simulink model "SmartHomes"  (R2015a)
settings: Solver=ode45  StartTime=0.0  StopTime=87600  RelTol=1e-3
model workspace (MAT data in the model file):
  batteryCostPerKwh = 500
  batterySize = 7
  oneTimeCost = 1000
  costPerKwhFromUtility = 0.2881
  annualChangeOfCostPerKwhFromUtility = 3.4
  solarPanelEfficiency = 16
  costPerKwhBoughtFromBattery = 0.18
  compensationPerKwhSoldToBattery = 0.18
  numberOfHouses = 1
  MCOS : class17 (value not decoded)
  MCOS : class17 (value not decoded)
undefined symbols (not defined in the file or in its folder): csvread, randi
libraries: simulink x19

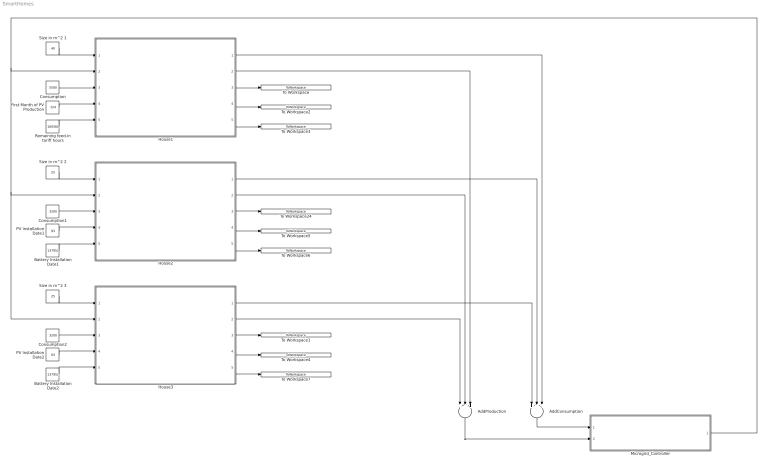
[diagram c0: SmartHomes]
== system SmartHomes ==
  AddConsumption : Sum  Inputs=+++
  AddProduction : Sum  Inputs=+++
  Battery Installation Date1 : Constant  Value=137952
  Battery Installation Date2 : Constant  Value=137952
  Consumption : Constant  Value=5500
  Consumption1 : Constant  Value=3200
  Consumption2 : Constant  Value=3200
  First Month of PV Production : Constant  Value=124
  House1 : Subsystem
  House2 : Subsystem
  House3 : Subsystem
  Microgrid_Controller : Subsystem
  PV Installation Date1 : Constant  Value=93
  PV Installation Date2 : Constant  Value=93
  Remaining feed-in tariff hours : Constant  Value=160560
  Size in m^2 1 : Constant  Value=40
  Size in m^2 2 : Constant  Value=25
  Size in m^2 3 : Constant  Value=25
  To Workspace : ToWorkspace  VariableName=merged_amortisation_house1  SaveFormat=Timeseries  SampleTime=-1
  To Workspace1 : ToWorkspace  VariableName=merged_amortisation_house  SaveFormat=Timeseries  SampleTime=-1
  To Workspace2 : ToWorkspace  VariableName=split_amortisation_house1  SaveFormat=Timeseries  SampleTime=-1
  To Workspace24 : ToWorkspace  VariableName=merged_amortisation_house2  SaveFormat=Timeseries  SampleTime=-1
  To Workspace3 : ToWorkspace  VariableName=net_sale_gradiant_house1  SaveFormat=Timeseries  SampleTime=-1
  To Workspace4 : ToWorkspace  VariableName=split_amortisation_house  SaveFormat=Timeseries  SampleTime=-1
  To Workspace5 : ToWorkspace  VariableName=split_amortisation_house2  SaveFormat=Timeseries  SampleTime=-1
  To Workspace6 : ToWorkspace  VariableName=net_sale_gradiant_house2  SaveFormat=Timeseries  SampleTime=-1
  To Workspace7 : ToWorkspace  VariableName=net_sale_gradiant_house  SaveFormat=Timeseries  SampleTime=-1
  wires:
  Size in m^2 1/1 -> House1/1(Solar Panel Size m²)
  AddConsumption/1 -> Microgrid_Controller/1(Energy Consumption (kWh))
  Consumption/1 -> House1/3(Yearly Consumption (kWh))
  AddProduction/1 -> Microgrid_Controller/2(Energy Production (kWh))
  House1/3(Merged Amortisation) -> To Workspace/1
  House1/4(Split Amortisation) -> To Workspace2/1
  House2/4(Split Amortisation) -> To Workspace5/1
  House2/3(Merged Amortisation) -> To Workspace24/1
  Remaining feed-in tariff hours/1 -> House1/5(Hours of Feed-In Tariff Remaining)
  First Month of PV Production/1 -> House1/4(First Month of PV Production)
  House1/2(Effective Energy Production (kWh)) -> AddProduction/3
  House1/1(Effective Energy Consumption (kWh)) -> AddConsumption/3
  House1/5(Grid Sale Gradient) -> To Workspace3/1
  House2/5(Grid Sale Gradient) -> To Workspace6/1
  Size in m^2 2/1 -> House2/1(Solar Panel Size m²)
  Consumption1/1 -> House2/3(Yearly Consumption (kWh))
  Battery Installation Date1/1 -> House2/5(Hours of Feed-In Tariff Remaining)
  PV Installation Date1/1 -> House2/4(First Month of PV Production)
  House3/4(Split Amortisation) -> To Workspace4/1
  House3/3(Merged Amortisation) -> To Workspace1/1
  House3/5(Grid Sale Gradient) -> To Workspace7/1
  Size in m^2 3/1 -> House3/1(Solar Panel Size m²)
  Consumption2/1 -> House3/3(Yearly Consumption (kWh))
  Battery Installation Date2/1 -> House3/5(Hours of Feed-In Tariff Remaining)
  PV Installation Date2/1 -> House3/4(First Month of PV Production)
  Microgrid_Controller/1(Battery Status) -> House1/2(Battey Status), House3/2(Battey Status), House2/2(Battey Status)
  House2/1(Effective Energy Consumption (kWh)) -> AddConsumption/2
  House2/2(Effective Energy Production (kWh)) -> AddProduction/2
  House3/1(Effective Energy Consumption (kWh)) -> AddConsumption/1
  House3/2(Effective Energy Production (kWh)) -> AddProduction/1

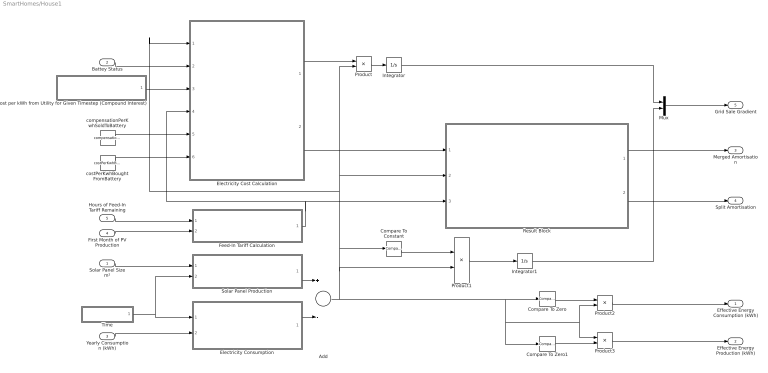
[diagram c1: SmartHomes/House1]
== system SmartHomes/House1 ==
  Solar Panel Size m² : Inport
  Battey Status : Inport  Port=2
  Yearly Consumption (kWh) : Inport  Port=3
  First Month of PV Production : Inport  Port=4
  Hours of Feed-In Tariff Remaining : Inport  Port=5
  Add : Sum  Inputs=+-
  Compare To Constant : simulink/Logic and Bit Operations/Compare To Constant  relop=>=  const=0  OutDataTypeStr=boolean
  Compare To Zero : simulink/Logic and Bit Operations/Compare To Zero  relop=<  OutDataTypeStr=boolean
  Compare To Zero1 : simulink/Logic and Bit Operations/Compare To Zero  relop=>=  OutDataTypeStr=boolean
  Cost per kWh from Utility for Given Timestep (Compound Interest) : Subsystem
  Electricity Consumption : Subsystem
  Electricity Cost Calculation : MATLAB Function  TreatAsAtomicUnit=on
  Feed-In Tariff Calculation : Subsystem
  Integrator : Integrator
  Integrator1 : Integrator
  Mux : Mux  Inputs=2
  Product{,1..3} (4 alike) : Product
  Result Block : Subsystem
  Solar Panel Production : Subsystem
  Time : Subsystem
  compensationPerKwhSoldToBattery : Constant  Value=compensationPerKwhSoldToBattery
  costPerKwhBoughtFromBattery : Constant  Value=costPerKwhBoughtFromBattery
  Effective Energy Consumption (kWh) : Outport
  Effective Energy Production (kWh) : Outport  Port=2
  Merged Amortisation : Outport  Port=3
  Split Amortisation : Outport  Port=4
  Grid Sale Gradient : Outport  Port=5
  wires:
  Time/1(Time in Hours % 8760) -> Solar Panel Production/2(Hour of Year), Electricity Consumption/1(Hour of Year)
  Solar Panel Size m²/1 -> Solar Panel Production/1(Solar Panel Size (m²))
  Yearly Consumption (kWh)/1 -> Electricity Consumption/2(Yearly Consumption (kWh))
  Product/1 -> Integrator/1
  Compare To Constant/1 -> Product1/1
  Product1/1 -> Integrator1/1
  Product2/1 -> Effective Energy Consumption (kWh)/1
  Product3/1 -> Effective Energy Production (kWh)/1
  Compare To Zero1/1 -> Product3/2
  Compare To Zero/1 -> Product2/1
  Battey Status/1 -> Electricity Cost Calculation/2(batteryStatus)
  costPerKwhBoughtFromBattery/1 -> Electricity Cost Calculation/6(internalBuyPrice)
  Cost per kWh from Utility for Given Timestep (Compound Interest)/1(Cost for kWh from Utility at Timestep) -> Electricity Cost Calculation/3(buyPrice)
  Electricity Cost Calculation/1(gridsaleAmount) -> Product/1
  Electricity Consumption/1(Consumtion kWh) -> Add/2
  Solar Panel Production/1(Solar Panel Production (kWh)) -> Add/1
  Add/1 -> Compare To Zero1/1, Product3/1, Product2/2, Compare To Zero/1, Product/2, Result Block/2(Effective Consumption / Production (kWh)), Electricity Cost Calculation/1(kWh), Compare To Constant/1, Product1/2
  Feed-In Tariff Calculation/1(Applcable Feed-In Tariff) -> Electricity Cost Calculation/4(sellPrice), Result Block/3(Applicable Feed-In Tariff (EUR))
  Result Block/1(House Result Merged) -> Merged Amortisation/1
  Result Block/2(House Result Split) -> Split Amortisation/1
  Integrator/1 -> Mux/1
  Integrator1/1 -> Mux/2
  Mux/1 -> Grid Sale Gradient/1
  Electricity Cost Calculation/2(cost) -> Result Block/1(Effective Cost of Electricity for Timestep (EUR))
  Hours of Feed-In Tariff Remaining/1 -> Feed-In Tariff Calculation/1(Hours of Feed-In Tariff Remaining)
  First Month of PV Production/1 -> Feed-In Tariff Calculation/2(First Month of PV Production)
  compensationPerKwhSoldToBattery/1 -> Electricity Cost Calculation/5(internalSellPrice)

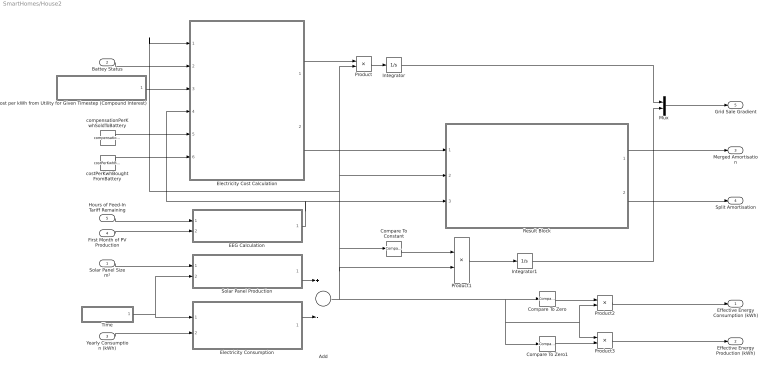
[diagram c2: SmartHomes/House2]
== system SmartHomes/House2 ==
  Solar Panel Size m² : Inport
  Battey Status : Inport  Port=2
  Yearly Consumption (kWh) : Inport  Port=3
  First Month of PV Production : Inport  Port=4
  Hours of Feed-In Tariff Remaining : Inport  Port=5
  Add : Sum  Inputs=+-
  Compare To Constant : simulink/Logic and Bit Operations/Compare To Constant  relop=>=  const=0  OutDataTypeStr=boolean
  Compare To Zero : simulink/Logic and Bit Operations/Compare To Zero  relop=<  OutDataTypeStr=boolean
  Compare To Zero1 : simulink/Logic and Bit Operations/Compare To Zero  relop=>=  OutDataTypeStr=boolean
  Cost per kWh from Utility for Given Timestep (Compound Interest) : Subsystem
  EEG Calculation : Subsystem
  Electricity Consumption : Subsystem
  Electricity Cost Calculation : MATLAB Function  TreatAsAtomicUnit=on
  Integrator : Integrator
  Integrator1 : Integrator
  Mux : Mux  Inputs=2
  Product{,1..3} (4 alike) : Product
  Result Block : Subsystem
  Solar Panel Production : Subsystem
  Time : Subsystem
  compensationPerKwhSoldToBattery : Constant  Value=compensationPerKwhSoldToBattery
  costPerKwhBoughtFromBattery : Constant  Value=costPerKwhBoughtFromBattery
  Effective Energy Consumption (kWh) : Outport
  Effective Energy Production (kWh) : Outport  Port=2
  Merged Amortisation : Outport  Port=3
  Split Amortisation : Outport  Port=4
  Grid Sale Gradient : Outport  Port=5
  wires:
  Time/1(Time in Hours % 8760) -> Solar Panel Production/2(Hour of Year), Electricity Consumption/1(Hour of Year)
  Solar Panel Size m²/1 -> Solar Panel Production/1(Solar Panel Size (m²))
  Yearly Consumption (kWh)/1 -> Electricity Consumption/2(Yearly Consumption (kWh))
  Product/1 -> Integrator/1
  Compare To Constant/1 -> Product1/1
  Product1/1 -> Integrator1/1
  Product2/1 -> Effective Energy Consumption (kWh)/1
  Product3/1 -> Effective Energy Production (kWh)/1
  Compare To Zero1/1 -> Product3/2
  Compare To Zero/1 -> Product2/1
  Battey Status/1 -> Electricity Cost Calculation/2(batteryStatus)
  costPerKwhBoughtFromBattery/1 -> Electricity Cost Calculation/6(internalBuyPrice)
  Cost per kWh from Utility for Given Timestep (Compound Interest)/1(Cost for kWh from Utility at Timestep) -> Electricity Cost Calculation/3(buyPrice)
  Electricity Cost Calculation/1(gridsaleAmount) -> Product/1
  Electricity Consumption/1(Consumtion kWh) -> Add/2
  Solar Panel Production/1(Solar Panel Production (kWh)) -> Add/1
  Add/1 -> Compare To Zero1/1, Product3/1, Product2/2, Compare To Zero/1, Product/2, Result Block/2(Effective Consumption / Production (kWh)), Electricity Cost Calculation/1(kWh), Compare To Constant/1, Product1/2
  EEG Calculation/1(Applcable Feed-In Tariff) -> Electricity Cost Calculation/4(sellPrice), Result Block/3(Applicable Feed-In Tariff (EUR))
  Result Block/1(House Result Merged) -> Merged Amortisation/1
  Result Block/2(House Result Split) -> Split Amortisation/1
  Integrator/1 -> Mux/1
  Integrator1/1 -> Mux/2
  Mux/1 -> Grid Sale Gradient/1
  Electricity Cost Calculation/2(cost) -> Result Block/1(Effective Cost of Electricity for Timestep (EUR))
  Hours of Feed-In Tariff Remaining/1 -> EEG Calculation/1(Hours of Feed-In Tariff Remaining)
  First Month of PV Production/1 -> EEG Calculation/2(First Month of PV Production)
  compensationPerKwhSoldToBattery/1 -> Electricity Cost Calculation/5(internalSellPrice)

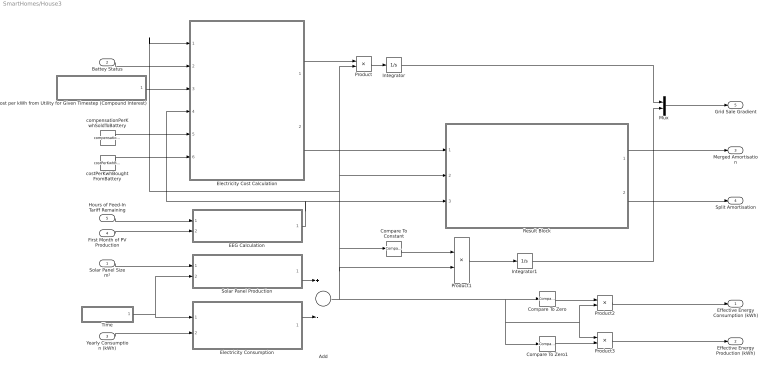
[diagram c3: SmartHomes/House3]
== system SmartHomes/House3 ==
  Solar Panel Size m² : Inport
  Battey Status : Inport  Port=2
  Yearly Consumption (kWh) : Inport  Port=3
  First Month of PV Production : Inport  Port=4
  Hours of Feed-In Tariff Remaining : Inport  Port=5
  Add : Sum  Inputs=+-
  Compare To Constant : simulink/Logic and Bit Operations/Compare To Constant  relop=>=  const=0  OutDataTypeStr=boolean
  Compare To Zero : simulink/Logic and Bit Operations/Compare To Zero  relop=<  OutDataTypeStr=boolean
  Compare To Zero1 : simulink/Logic and Bit Operations/Compare To Zero  relop=>=  OutDataTypeStr=boolean
  Cost per kWh from Utility for Given Timestep (Compound Interest) : Subsystem
  EEG Calculation : Subsystem
  Electricity Consumption : Subsystem
  Electricity Cost Calculation : MATLAB Function  TreatAsAtomicUnit=on
  Integrator : Integrator
  Integrator1 : Integrator
  Mux : Mux  Inputs=2
  Product{,1..3} (4 alike) : Product
  Result Block : Subsystem
  Solar Panel Production : Subsystem
  Time : Subsystem
  compensationPerKwhSoldToBattery : Constant  Value=compensationPerKwhSoldToBattery
  costPerKwhBoughtFromBattery : Constant  Value=costPerKwhBoughtFromBattery
  Effective Energy Consumption (kWh) : Outport
  Effective Energy Production (kWh) : Outport  Port=2
  Merged Amortisation : Outport  Port=3
  Split Amortisation : Outport  Port=4
  Grid Sale Gradient : Outport  Port=5
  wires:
  Time/1(Time in Hours % 8760) -> Solar Panel Production/2(Hour of Year), Electricity Consumption/1(Hour of Year)
  Solar Panel Size m²/1 -> Solar Panel Production/1(Solar Panel Size (m²))
  Yearly Consumption (kWh)/1 -> Electricity Consumption/2(Yearly Consumption (kWh))
  Product/1 -> Integrator/1
  Compare To Constant/1 -> Product1/1
  Product1/1 -> Integrator1/1
  Product2/1 -> Effective Energy Consumption (kWh)/1
  Product3/1 -> Effective Energy Production (kWh)/1
  Compare To Zero1/1 -> Product3/2
  Compare To Zero/1 -> Product2/1
  Battey Status/1 -> Electricity Cost Calculation/2(batteryStatus)
  costPerKwhBoughtFromBattery/1 -> Electricity Cost Calculation/6(internalBuyPrice)
  Cost per kWh from Utility for Given Timestep (Compound Interest)/1(Cost for kWh from Utility at Timestep) -> Electricity Cost Calculation/3(buyPrice)
  Electricity Cost Calculation/1(gridsaleAmount) -> Product/1
  Electricity Consumption/1(Consumtion kWh) -> Add/2
  Solar Panel Production/1(Solar Panel Production (kWh)) -> Add/1
  Add/1 -> Compare To Zero1/1, Product3/1, Product2/2, Compare To Zero/1, Product/2, Result Block/2(Effective Consumption / Production (kWh)), Electricity Cost Calculation/1(kWh), Compare To Constant/1, Product1/2
  EEG Calculation/1(Applcable Feed-In Tariff) -> Electricity Cost Calculation/4(sellPrice), Result Block/3(Applicable Feed-In Tariff (EUR))
  Result Block/1(House Result Merged) -> Merged Amortisation/1
  Result Block/2(House Result Split) -> Split Amortisation/1
  Integrator/1 -> Mux/1
  Integrator1/1 -> Mux/2
  Mux/1 -> Grid Sale Gradient/1
  Electricity Cost Calculation/2(cost) -> Result Block/1(Effective Cost of Electricity for Timestep (EUR))
  Hours of Feed-In Tariff Remaining/1 -> EEG Calculation/1(Hours of Feed-In Tariff Remaining)
  First Month of PV Production/1 -> EEG Calculation/2(First Month of PV Production)
  compensationPerKwhSoldToBattery/1 -> Electricity Cost Calculation/5(internalSellPrice)

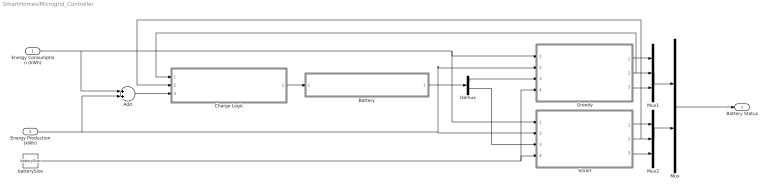
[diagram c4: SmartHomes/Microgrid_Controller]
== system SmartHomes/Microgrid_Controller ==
  Energy Consumption (kWh) : Inport
  Energy Production (kWh) : Inport  Port=2
  Add : Sum
  Battery : Subsystem
  Charge Logic : Subsystem
  Demux : Demux  Outputs=2
  Greedy : MATLAB Function  TreatAsAtomicUnit=on
  Mux : Mux  Inputs=2
  Mux1 : Mux  Inputs=3
  Mux2 : Mux  Inputs=3
  Smart : MATLAB Function  TreatAsAtomicUnit=on
  batterySize : Constant  Value=batterySize
  Battery Status : Outport
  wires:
  Charge Logic/1(Charge (kw/h)) -> Battery/1(Charge Amount (kWh))
  Mux/1 -> Battery Status/1
  batterySize/1 -> Smart/4(batterySize), Greedy/4(batterySize)
  Add/1 -> Charge Logic/3(Net Energy Amount (kWh))
  Demux/2 -> Smart/3(currentBatteryCharge)
  Demux/1 -> Greedy/3(currentBatteryCharge)
  Energy Consumption (kWh)/1 -> Greedy/1(Consumption), Smart/1(Consumption), Add/1
  Energy Production (kWh)/1 -> Smart/2(Production), Greedy/2(Production), Add/2
  Greedy/2(p2) -> Mux1/2, Charge Logic/1(Internal Trade Percentage - Greedy)
  Greedy/3(p3) -> Mux1/3
  Greedy/1(p1) -> Mux1/1
  Mux1/1 -> Mux/1
  Smart/1(p1) -> Mux2/1
  Smart/2(p2) -> Charge Logic/2(Internal Trade Percentage - Smart), Mux2/2
  Smart/3(p3) -> Mux2/3
  Mux2/1 -> Mux/2
  Battery/1(Current Battery Charge (kWh)) -> Demux/1

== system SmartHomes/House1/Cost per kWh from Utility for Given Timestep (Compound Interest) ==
  Calculate Year of Simulation Step : Subsystem
  Compound Interest for Cost per kWh from Utility (EUR) : Fcn  Expr=u(2) * (1 + u(3) / 100) ^ u(1)
  Mux1 : Mux  Inputs=3
  annualChangeOfCostPerKwhFromUtility : Constant  Value=annualChangeOfCostPerKwhFromUtility
  costPerKwhFromUtility : Constant  Value=costPerKwhFromUtility
  Cost for kWh from Utility at Timestep : Outport
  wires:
  Mux1/1 -> Compound Interest for Cost per kWh from Utility (EUR)/1
  annualChangeOfCostPerKwhFromUtility/1 -> Mux1/3
  Calculate Year of Simulation Step/1(Out1) -> Mux1/1
  Compound Interest for Cost per kWh from Utility (EUR)/1 -> Cost for kWh from Utility at Timestep/1
  costPerKwhFromUtility/1 -> Mux1/2

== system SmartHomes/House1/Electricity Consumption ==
  Hour of Year : Inport
  Yearly Consumption (kWh) : Inport  Port=2
  Add : Sum
  Consumption per Hour of Day (kWh) : LookupNDDirect  NumberOfTableDimensions=1  Table=csvread('raw_data/netherlands_consumption_e1a.csv');  DiagnosticForOutOfRangeInput=Error
  Product : Product
  Saturation : Saturate  UpperLimit=5*10e-5  LowerLimit=-5*10e-5
  Variance : RandomNumber  Variance=0.00000000013014  Seed=randi(66666);  SampleTime=1
  Consumtion kWh : Outport
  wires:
  Add/1 -> Product/1
  Consumption per Hour of Day (kWh)/1 -> Add/1
  Hour of Year/1 -> Consumption per Hour of Day (kWh)/1
  Yearly Consumption (kWh)/1 -> Product/2
  Product/1 -> Consumtion kWh/1
  Variance/1 -> Saturation/1
  Saturation/1 -> Add/2

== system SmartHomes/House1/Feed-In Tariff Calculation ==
  Hours of Feed-In Tariff Remaining : Inport
  First Month of PV Production : Inport  Port=2
  Compare To Constant : simulink/Logic and Bit Operations/Compare To Constant  relop=>=  const=0  OutDataTypeStr=boolean
  Constant : Constant  Value=100
  Digtal Clock : DigitalClock
  Divide : Product  Inputs=*/
  EEG-Values : LookupNDDirect  NumberOfTableDimensions=1  Table=csvread('raw_data/feed-in_tariff_data.csv');  DiagnosticForOutOfRangeInput=Error
  Product : Product
  Subtract : Sum  Inputs=+-
  Applcable Feed-In Tariff : Outport
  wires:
  First Month of PV Production/1 -> EEG-Values/1
  Hours of Feed-In Tariff Remaining/1 -> Subtract/1
  Digtal Clock/1 -> Subtract/2
  Subtract/1 -> Compare To Constant/1
  Compare To Constant/1 -> Product/1
  EEG-Values/1 -> Product/2
  Divide/1 -> Applcable Feed-In Tariff/1
  Product/1 -> Divide/1
  Constant/1 -> Divide/2

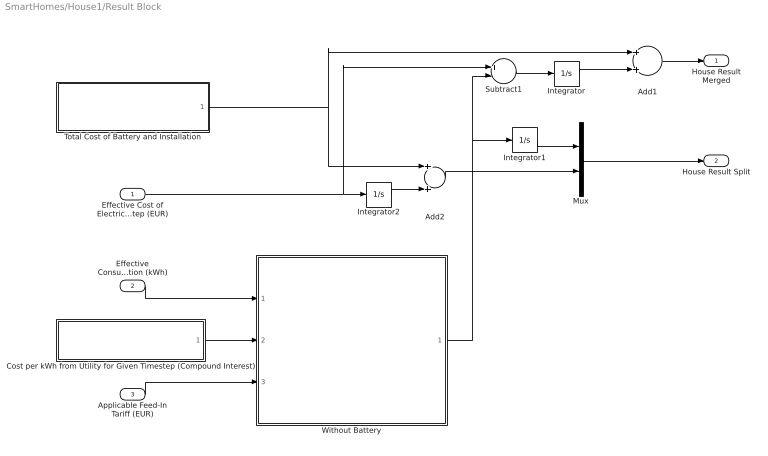
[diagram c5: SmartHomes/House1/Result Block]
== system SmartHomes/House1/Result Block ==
  Effective Cost of Electricity for Timestep (EUR) : Inport
  Effective Consumption / Production (kWh) : Inport  Port=2
  Applicable Feed-In Tariff (EUR) : Inport  Port=3
  Add1 : Sum
  Add2 : Sum
  Cost per kWh from Utility for Given Timestep (Compound Interest) : Subsystem
  Integrator : Integrator
  Integrator1 : Integrator
  Integrator2 : Integrator
  Mux : Mux  Inputs=2
  Subtract1 : Sum  Inputs=+-
  Total Cost of Battery and Installation : Subsystem
  Without Battery : Subsystem
  House Result Merged : Outport
  House Result Split : Outport  Port=2
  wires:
  Applicable Feed-In Tariff (EUR)/1 -> Without Battery/3(Sell Price to Utility (EUR))
  Subtract1/1 -> Integrator/1
  Effective Cost of Electricity for Timestep (EUR)/1 -> Subtract1/1, Integrator2/1
  Add1/1 -> House Result Merged/1
  Effective Consumption / Production (kWh)/1 -> Without Battery/1(Effective Consumption / Production (kWh))
  Integrator/1 -> Add1/2
  Mux/1 -> House Result Split/1
  Integrator1/1 -> Mux/1
  Integrator2/1 -> Add2/2
  Add2/1 -> Mux/2
  Total Cost of Battery and Installation/1(Total Cost of Battery and Installation) -> Add1/1, Add2/1
  Cost per kWh from Utility for Given Timestep (Compound Interest)/1(Cost per kWh from Utility at Timestep) -> Without Battery/2(Cost per kWh from Utility (EUR))
  Without Battery/1(Result EUR) -> Integrator1/1, Subtract1/2

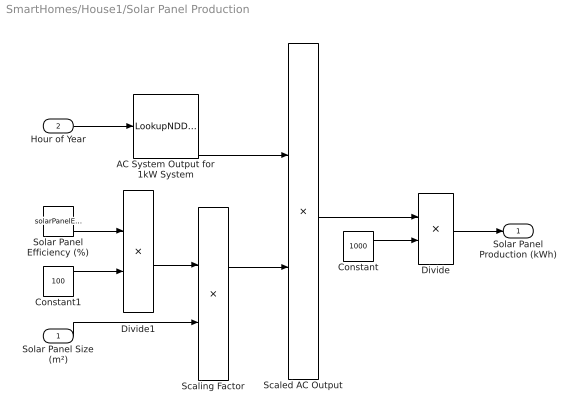
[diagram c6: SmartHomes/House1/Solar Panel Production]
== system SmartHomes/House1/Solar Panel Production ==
  Solar Panel Size (m²) : Inport
  Hour of Year : Inport  Port=2
  AC System Output for 1kW System : LookupNDDirect  NumberOfTableDimensions=1  Table=csvread('raw_data/pvwatts_data_1kwp.csv');  DiagnosticForOutOfRangeInput=Error
  Constant : Constant  Value=1000
  Constant1 : Constant  Value=100
  Divide : Product  Inputs=*/
  Divide1 : Product  Inputs=*/
  Scaled AC Output : Product
  Scaling Factor : Product
  Solar Panel Efficiency (%) : Constant  Value=solarPanelEfficiency
  Solar Panel Production (kWh) : Outport
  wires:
  Solar Panel Efficiency (%)/1 -> Divide1/1
  Scaling Factor/1 -> Scaled AC Output/2
  AC System Output for 1kW System/1 -> Scaled AC Output/1
  Solar Panel Size (m²)/1 -> Scaling Factor/2
  Hour of Year/1 -> AC System Output for 1kW System/1
  Scaled AC Output/1 -> Divide/1
  Constant/1 -> Divide/2
  Divide/1 -> Solar Panel Production (kWh)/1
  Constant1/1 -> Divide1/2
  Divide1/1 -> Scaling Factor/1

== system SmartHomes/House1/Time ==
  Digtal Clock : DigitalClock
  Hours in a Year : Constant  Value=8760
  Modulo : Math  Operator=mod
  Time in Hours % 8760 : Outport
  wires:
  Digtal Clock/1 -> Modulo/1
  Hours in a Year/1 -> Modulo/2
  Modulo/1 -> Time in Hours % 8760/1

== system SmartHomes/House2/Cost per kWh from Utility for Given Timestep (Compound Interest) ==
  Calculate Year of Simulation Step : Subsystem
  Compound Interest for Cost per kWh from Utility (EUR) : Fcn  Expr=u(2) * (1 + u(3) / 100) ^ u(1)
  Mux1 : Mux  Inputs=3
  annualChangeOfCostPerKwhFromUtility : Constant  Value=annualChangeOfCostPerKwhFromUtility
  costPerKwhFromUtility : Constant  Value=costPerKwhFromUtility
  Cost for kWh from Utility at Timestep : Outport
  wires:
  Mux1/1 -> Compound Interest for Cost per kWh from Utility (EUR)/1
  annualChangeOfCostPerKwhFromUtility/1 -> Mux1/3
  Calculate Year of Simulation Step/1(Out1) -> Mux1/1
  Compound Interest for Cost per kWh from Utility (EUR)/1 -> Cost for kWh from Utility at Timestep/1
  costPerKwhFromUtility/1 -> Mux1/2

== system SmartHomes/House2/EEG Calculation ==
  Hours of Feed-In Tariff Remaining : Inport
  First Month of PV Production : Inport  Port=2
  Compare To Constant : simulink/Logic and Bit Operations/Compare To Constant  relop=>=  const=0  OutDataTypeStr=boolean
  Constant : Constant  Value=100
  Digtal Clock : DigitalClock
  Divide : Product  Inputs=*/
  EEG-Values : LookupNDDirect  NumberOfTableDimensions=1  Table=csvread('raw_data/feed-in_tariff_data.csv');  DiagnosticForOutOfRangeInput=Error
  Product : Product
  Subtract : Sum  Inputs=+-
  Applcable Feed-In Tariff : Outport
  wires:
  First Month of PV Production/1 -> EEG-Values/1
  Hours of Feed-In Tariff Remaining/1 -> Subtract/1
  Digtal Clock/1 -> Subtract/2
  Subtract/1 -> Compare To Constant/1
  Compare To Constant/1 -> Product/1
  EEG-Values/1 -> Product/2
  Divide/1 -> Applcable Feed-In Tariff/1
  Product/1 -> Divide/1
  Constant/1 -> Divide/2

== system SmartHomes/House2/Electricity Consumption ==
  Hour of Year : Inport
  Yearly Consumption (kWh) : Inport  Port=2
  Add : Sum
  Consumption per Hour of Day (kWh) : LookupNDDirect  NumberOfTableDimensions=1  Table=csvread('raw_data/netherlands_consumption_e1a.csv');  DiagnosticForOutOfRangeInput=Error
  Product : Product
  Saturation : Saturate  UpperLimit=5*10e-5  LowerLimit=-5*10e-5
  Variance : RandomNumber  Variance=0.00000000013014  Seed=randi(66666);  SampleTime=1
  Consumtion kWh : Outport
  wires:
  Add/1 -> Product/1
  Consumption per Hour of Day (kWh)/1 -> Add/1
  Hour of Year/1 -> Consumption per Hour of Day (kWh)/1
  Yearly Consumption (kWh)/1 -> Product/2
  Product/1 -> Consumtion kWh/1
  Variance/1 -> Saturation/1
  Saturation/1 -> Add/2

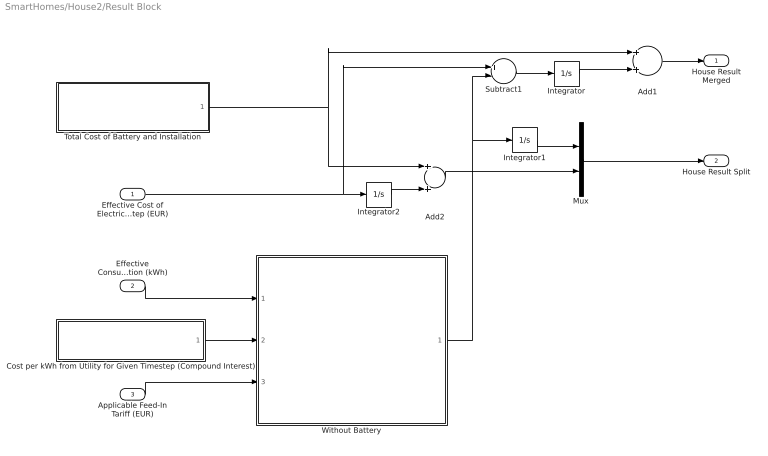
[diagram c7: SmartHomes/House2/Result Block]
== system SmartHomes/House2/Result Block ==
  Effective Cost of Electricity for Timestep (EUR) : Inport
  Effective Consumption / Production (kWh) : Inport  Port=2
  Applicable Feed-In Tariff (EUR) : Inport  Port=3
  Add1 : Sum
  Add2 : Sum
  Cost per kWh from Utility for Given Timestep (Compound Interest) : Subsystem
  Integrator : Integrator
  Integrator1 : Integrator
  Integrator2 : Integrator
  Mux : Mux  Inputs=2
  Subtract1 : Sum  Inputs=+-
  Total Cost of Battery and Installation : Subsystem
  Without Battery : Subsystem
  House Result Merged : Outport
  House Result Split : Outport  Port=2
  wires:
  Applicable Feed-In Tariff (EUR)/1 -> Without Battery/3(Sell Price to Utility (EUR))
  Subtract1/1 -> Integrator/1
  Effective Cost of Electricity for Timestep (EUR)/1 -> Subtract1/1, Integrator2/1
  Add1/1 -> House Result Merged/1
  Effective Consumption / Production (kWh)/1 -> Without Battery/1(Effective Consumption / Production (kWh))
  Integrator/1 -> Add1/2
  Mux/1 -> House Result Split/1
  Integrator1/1 -> Mux/1
  Integrator2/1 -> Add2/2
  Add2/1 -> Mux/2
  Total Cost of Battery and Installation/1(Total Cost of Battery and Installation) -> Add1/1, Add2/1
  Cost per kWh from Utility for Given Timestep (Compound Interest)/1(Cost per kWh from Utility at Timestep) -> Without Battery/2(Cost per kWh from Utility (EUR))
  Without Battery/1(Result EUR) -> Integrator1/1, Subtract1/2

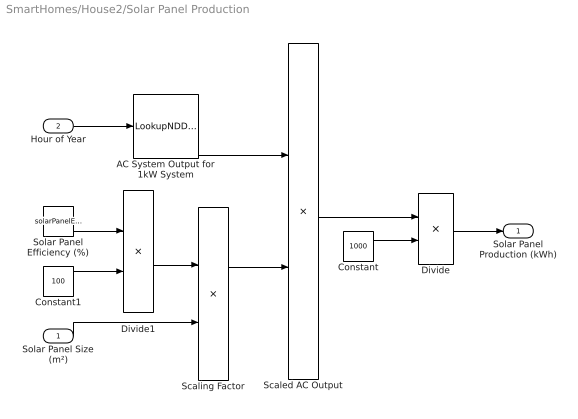
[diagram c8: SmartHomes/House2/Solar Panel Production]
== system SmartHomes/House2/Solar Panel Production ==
  Solar Panel Size (m²) : Inport
  Hour of Year : Inport  Port=2
  AC System Output for 1kW System : LookupNDDirect  NumberOfTableDimensions=1  Table=csvread('raw_data/pvwatts_data_1kwp.csv');  DiagnosticForOutOfRangeInput=Error
  Constant : Constant  Value=1000
  Constant1 : Constant  Value=100
  Divide : Product  Inputs=*/
  Divide1 : Product  Inputs=*/
  Scaled AC Output : Product
  Scaling Factor : Product
  Solar Panel Efficiency (%) : Constant  Value=solarPanelEfficiency
  Solar Panel Production (kWh) : Outport
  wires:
  Solar Panel Efficiency (%)/1 -> Divide1/1
  Scaling Factor/1 -> Scaled AC Output/2
  AC System Output for 1kW System/1 -> Scaled AC Output/1
  Solar Panel Size (m²)/1 -> Scaling Factor/2
  Hour of Year/1 -> AC System Output for 1kW System/1
  Scaled AC Output/1 -> Divide/1
  Constant/1 -> Divide/2
  Divide/1 -> Solar Panel Production (kWh)/1
  Constant1/1 -> Divide1/2
  Divide1/1 -> Scaling Factor/1

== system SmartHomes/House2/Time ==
  Digtal Clock : DigitalClock
  Hours in a Year : Constant  Value=8760
  Modulo : Math  Operator=mod
  Time in Hours % 8760 : Outport
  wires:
  Digtal Clock/1 -> Modulo/1
  Hours in a Year/1 -> Modulo/2
  Modulo/1 -> Time in Hours % 8760/1

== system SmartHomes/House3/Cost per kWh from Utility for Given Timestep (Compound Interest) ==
  Calculate Year of Simulation Step : Subsystem
  Compound Interest for Cost per kWh from Utility (EUR) : Fcn  Expr=u(2) * (1 + u(3) / 100) ^ u(1)
  Mux1 : Mux  Inputs=3
  annualChangeOfCostPerKwhFromUtility : Constant  Value=annualChangeOfCostPerKwhFromUtility
  costPerKwhFromUtility : Constant  Value=costPerKwhFromUtility
  Cost for kWh from Utility at Timestep : Outport
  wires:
  Mux1/1 -> Compound Interest for Cost per kWh from Utility (EUR)/1
  annualChangeOfCostPerKwhFromUtility/1 -> Mux1/3
  Calculate Year of Simulation Step/1(Out1) -> Mux1/1
  Compound Interest for Cost per kWh from Utility (EUR)/1 -> Cost for kWh from Utility at Timestep/1
  costPerKwhFromUtility/1 -> Mux1/2

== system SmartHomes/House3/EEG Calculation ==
  Hours of Feed-In Tariff Remaining : Inport
  First Month of PV Production : Inport  Port=2
  Compare To Constant : simulink/Logic and Bit Operations/Compare To Constant  relop=>=  const=0  OutDataTypeStr=boolean
  Constant : Constant  Value=100
  Digtal Clock : DigitalClock
  Divide : Product  Inputs=*/
  EEG-Values : LookupNDDirect  NumberOfTableDimensions=1  Table=csvread('raw_data/feed-in_tariff_data.csv');  DiagnosticForOutOfRangeInput=Error
  Product : Product
  Subtract : Sum  Inputs=+-
  Applcable Feed-In Tariff : Outport
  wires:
  First Month of PV Production/1 -> EEG-Values/1
  Hours of Feed-In Tariff Remaining/1 -> Subtract/1
  Digtal Clock/1 -> Subtract/2
  Subtract/1 -> Compare To Constant/1
  Compare To Constant/1 -> Product/1
  EEG-Values/1 -> Product/2
  Divide/1 -> Applcable Feed-In Tariff/1
  Product/1 -> Divide/1
  Constant/1 -> Divide/2

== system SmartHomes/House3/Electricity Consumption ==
  Hour of Year : Inport
  Yearly Consumption (kWh) : Inport  Port=2
  Add : Sum
  Consumption per Hour of Day (kWh) : LookupNDDirect  NumberOfTableDimensions=1  Table=csvread('raw_data/netherlands_consumption_e1a.csv');  DiagnosticForOutOfRangeInput=Error
  Product : Product
  Saturation : Saturate  UpperLimit=5*10e-5  LowerLimit=-5*10e-5
  Variance : RandomNumber  Variance=0.00000000013014  Seed=randi(66666);  SampleTime=1
  Consumtion kWh : Outport
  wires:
  Add/1 -> Product/1
  Consumption per Hour of Day (kWh)/1 -> Add/1
  Hour of Year/1 -> Consumption per Hour of Day (kWh)/1
  Yearly Consumption (kWh)/1 -> Product/2
  Product/1 -> Consumtion kWh/1
  Variance/1 -> Saturation/1
  Saturation/1 -> Add/2

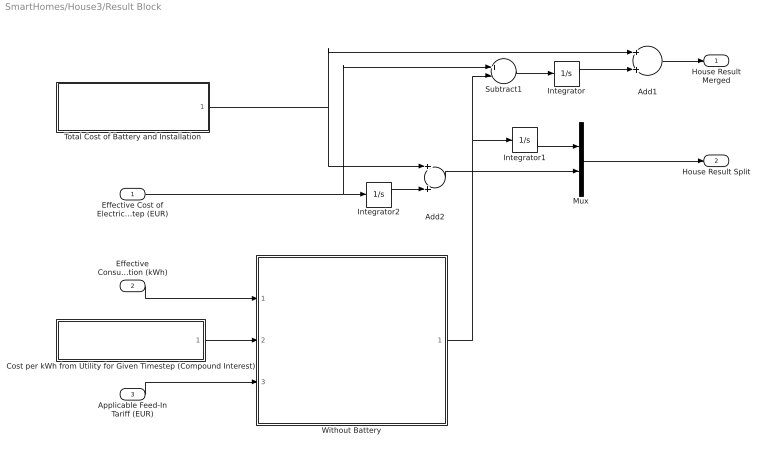
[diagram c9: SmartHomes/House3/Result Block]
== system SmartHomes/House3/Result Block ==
  Effective Cost of Electricity for Timestep (EUR) : Inport
  Effective Consumption / Production (kWh) : Inport  Port=2
  Applicable Feed-In Tariff (EUR) : Inport  Port=3
  Add1 : Sum
  Add2 : Sum
  Cost per kWh from Utility for Given Timestep (Compound Interest) : Subsystem
  Integrator : Integrator
  Integrator1 : Integrator
  Integrator2 : Integrator
  Mux : Mux  Inputs=2
  Subtract1 : Sum  Inputs=+-
  Total Cost of Battery and Installation : Subsystem
  Without Battery : Subsystem
  House Result Merged : Outport
  House Result Split : Outport  Port=2
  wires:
  Applicable Feed-In Tariff (EUR)/1 -> Without Battery/3(Sell Price to Utility (EUR))
  Subtract1/1 -> Integrator/1
  Effective Cost of Electricity for Timestep (EUR)/1 -> Subtract1/1, Integrator2/1
  Add1/1 -> House Result Merged/1
  Effective Consumption / Production (kWh)/1 -> Without Battery/1(Effective Consumption / Production (kWh))
  Integrator/1 -> Add1/2
  Mux/1 -> House Result Split/1
  Integrator1/1 -> Mux/1
  Integrator2/1 -> Add2/2
  Add2/1 -> Mux/2
  Total Cost of Battery and Installation/1(Total Cost of Battery and Installation) -> Add1/1, Add2/1
  Cost per kWh from Utility for Given Timestep (Compound Interest)/1(Cost per kWh from Utility at Timestep) -> Without Battery/2(Cost per kWh from Utility (EUR))
  Without Battery/1(Result EUR) -> Integrator1/1, Subtract1/2

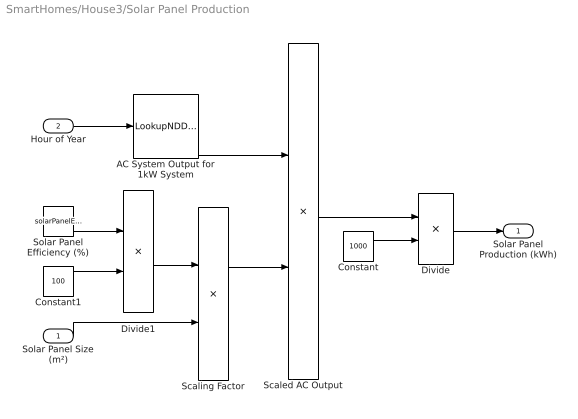
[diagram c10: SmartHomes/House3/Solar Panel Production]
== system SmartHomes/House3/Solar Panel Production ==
  Solar Panel Size (m²) : Inport
  Hour of Year : Inport  Port=2
  AC System Output for 1kW System : LookupNDDirect  NumberOfTableDimensions=1  Table=csvread('raw_data/pvwatts_data_1kwp.csv');  DiagnosticForOutOfRangeInput=Error
  Constant : Constant  Value=1000
  Constant1 : Constant  Value=100
  Divide : Product  Inputs=*/
  Divide1 : Product  Inputs=*/
  Scaled AC Output : Product
  Scaling Factor : Product
  Solar Panel Efficiency (%) : Constant  Value=solarPanelEfficiency
  Solar Panel Production (kWh) : Outport
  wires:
  Solar Panel Efficiency (%)/1 -> Divide1/1
  Scaling Factor/1 -> Scaled AC Output/2
  AC System Output for 1kW System/1 -> Scaled AC Output/1
  Solar Panel Size (m²)/1 -> Scaling Factor/2
  Hour of Year/1 -> AC System Output for 1kW System/1
  Scaled AC Output/1 -> Divide/1
  Constant/1 -> Divide/2
  Divide/1 -> Solar Panel Production (kWh)/1
  Constant1/1 -> Divide1/2
  Divide1/1 -> Scaling Factor/1

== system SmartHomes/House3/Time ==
  Digtal Clock : DigitalClock
  Hours in a Year : Constant  Value=8760
  Modulo : Math  Operator=mod
  Time in Hours % 8760 : Outport
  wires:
  Digtal Clock/1 -> Modulo/1
  Hours in a Year/1 -> Modulo/2
  Modulo/1 -> Time in Hours % 8760/1

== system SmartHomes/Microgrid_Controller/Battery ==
  Charge Amount (kWh) : Inport
  Battery : Integrator
  To Workspace : ToWorkspace  VariableName=neighbourhood_battery_charge_over_time  SaveFormat=Timeseries  SampleTime=-1
  Current Battery Charge (kWh) : Outport
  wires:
  Battery/1 -> Current Battery Charge (kWh)/1, To Workspace/1
  Charge Amount (kWh)/1 -> Battery/1

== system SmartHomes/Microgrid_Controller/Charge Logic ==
  Internal Trade Percentage - Greedy : Inport
  Internal Trade Percentage - Smart : Inport  Port=2
  Net Energy Amount (kWh) : Inport  Port=3
  Compare To Constant : simulink/Logic and Bit Operations/Compare To Constant  relop===  const=1  OutDataTypeStr=boolean
  Mux : Mux  Inputs=2
  Product : Product
  Charge (kw/h) : Outport
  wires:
  Net Energy Amount (kWh)/1 -> Product/1
  Product/1 -> Charge (kw/h)/1
  Internal Trade Percentage - Greedy/1 -> Mux/1
  Mux/1 -> Compare To Constant/1
  Internal Trade Percentage - Smart/1 -> Mux/2
  Compare To Constant/1 -> Product/2

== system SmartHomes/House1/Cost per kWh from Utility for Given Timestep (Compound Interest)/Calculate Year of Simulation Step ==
  Digital Clock : DigitalClock
  Fcn : Fcn  Expr=floor(u/8760)
  Out1 : Outport
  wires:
  Fcn/1 -> Out1/1
  Digital Clock/1 -> Fcn/1

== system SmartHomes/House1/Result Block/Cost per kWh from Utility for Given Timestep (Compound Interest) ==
  Calculate Year of Simulation Step : Subsystem
  Compound Interest for Cost per kWh from Utility (EUR) : Fcn  Expr=u(2) * (1 + u(3) / 100) ^ u(1)
  Mux1 : Mux  Inputs=3
  annualChangeOfCostPerKwhFromUtility : Constant  Value=annualChangeOfCostPerKwhFromUtility
  costPerKwhFromUtility : Constant  Value=costPerKwhFromUtility
  Cost per kWh from Utility at Timestep : Outport
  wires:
  Mux1/1 -> Compound Interest for Cost per kWh from Utility (EUR)/1
  annualChangeOfCostPerKwhFromUtility/1 -> Mux1/3
  Calculate Year of Simulation Step/1(Out1) -> Mux1/1
  Compound Interest for Cost per kWh from Utility (EUR)/1 -> Cost per kWh from Utility at Timestep/1
  costPerKwhFromUtility/1 -> Mux1/2

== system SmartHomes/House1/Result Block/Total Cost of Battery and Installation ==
  Add : Sum
  Constant : Constant  Value=-1
  Divide : Product  Inputs=*/
  Number of Houses : Constant  Value=numberOfHouses
  Product : Product
  Product1 : Product
  batteryCostPerKwh : Constant  Value=batteryCostPerKwh
  "batterySize " : Constant  Value=batterySize
  oneTimeCost : Constant  Value=oneTimeCost
  Total Cost of Battery and Installation : Outport
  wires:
  Constant/1 -> Product/1
  oneTimeCost/1 -> Add/1
  Number of Houses/1 -> Divide/2
  Add/1 -> Divide/1
  Divide/1 -> Product/2
  "batterySize "/1 -> Product1/2
  Product/1 -> Total Cost of Battery and Installation/1
  batteryCostPerKwh/1 -> Product1/1
  Product1/1 -> Add/2

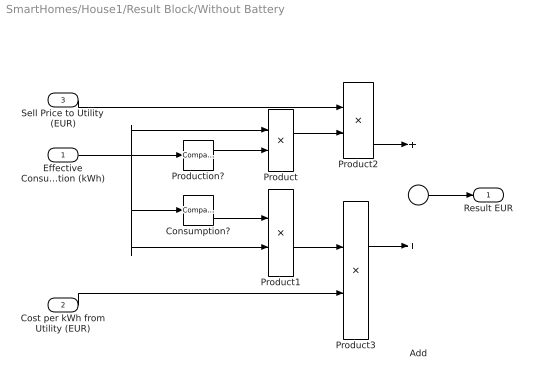
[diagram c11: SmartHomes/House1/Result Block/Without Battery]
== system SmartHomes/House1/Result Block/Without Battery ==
  Effective Consumption / Production (kWh) : Inport
  Cost per kWh from Utility (EUR) : Inport  Port=2
  Sell Price to Utility (EUR) : Inport  Port=3
  Add : Sum
  Consumption? : simulink/Logic and Bit Operations/Compare To Zero  relop=<  OutDataTypeStr=boolean
  Product{,1..3} (4 alike) : Product
  Production? : simulink/Logic and Bit Operations/Compare To Zero  relop=>=  OutDataTypeStr=boolean
  Result EUR : Outport
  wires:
  Effective Consumption / Production (kWh)/1 -> Product/1, Product1/2, Consumption?/1, Production?/1
  Consumption?/1 -> Product1/1
  Production?/1 -> Product/2
  Product/1 -> Product2/2
  Sell Price to Utility (EUR)/1 -> Product2/1
  Product1/1 -> Product3/1
  Cost per kWh from Utility (EUR)/1 -> Product3/2
  Product3/1 -> Add/2
  Product2/1 -> Add/1
  Add/1 -> Result EUR/1

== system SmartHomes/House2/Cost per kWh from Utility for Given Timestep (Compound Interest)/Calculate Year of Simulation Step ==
  Digital Clock : DigitalClock
  Fcn : Fcn  Expr=floor(u/8760)
  Out1 : Outport
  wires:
  Fcn/1 -> Out1/1
  Digital Clock/1 -> Fcn/1

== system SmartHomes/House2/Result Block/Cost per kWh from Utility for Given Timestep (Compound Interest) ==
  Calculate Year of Simulation Step : Subsystem
  Compound Interest for Cost per kWh from Utility (EUR) : Fcn  Expr=u(2) * (1 + u(3) / 100) ^ u(1)
  Mux1 : Mux  Inputs=3
  annualChangeOfCostPerKwhFromUtility : Constant  Value=annualChangeOfCostPerKwhFromUtility
  costPerKwhFromUtility : Constant  Value=costPerKwhFromUtility
  Cost per kWh from Utility at Timestep : Outport
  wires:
  Mux1/1 -> Compound Interest for Cost per kWh from Utility (EUR)/1
  annualChangeOfCostPerKwhFromUtility/1 -> Mux1/3
  Calculate Year of Simulation Step/1(Out1) -> Mux1/1
  Compound Interest for Cost per kWh from Utility (EUR)/1 -> Cost per kWh from Utility at Timestep/1
  costPerKwhFromUtility/1 -> Mux1/2

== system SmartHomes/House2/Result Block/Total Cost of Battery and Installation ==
  Add : Sum
  Constant : Constant  Value=-1
  Divide : Product  Inputs=*/
  Number of Houses : Constant  Value=numberOfHouses
  Product : Product
  Product1 : Product
  batteryCostPerKwh : Constant  Value=batteryCostPerKwh
  "batterySize " : Constant  Value=batterySize
  oneTimeCost : Constant  Value=oneTimeCost
  Total Cost of Battery and Installation : Outport
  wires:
  Constant/1 -> Product/1
  oneTimeCost/1 -> Add/1
  Number of Houses/1 -> Divide/2
  Add/1 -> Divide/1
  Divide/1 -> Product/2
  "batterySize "/1 -> Product1/2
  Product/1 -> Total Cost of Battery and Installation/1
  batteryCostPerKwh/1 -> Product1/1
  Product1/1 -> Add/2

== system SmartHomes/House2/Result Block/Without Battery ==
  Effective Consumption / Production (kWh) : Inport
  Cost per kWh from Utility (EUR) : Inport  Port=2
  Sell Price to Utility (EUR) : Inport  Port=3
  Add : Sum
  Consumption? : simulink/Logic and Bit Operations/Compare To Zero  relop=<  OutDataTypeStr=boolean
  Product{,1..3} (4 alike) : Product
  Production? : simulink/Logic and Bit Operations/Compare To Zero  relop=>=  OutDataTypeStr=boolean
  Result EUR : Outport
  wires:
  Effective Consumption / Production (kWh)/1 -> Product/1, Product1/2, Consumption?/1, Production?/1
  Consumption?/1 -> Product1/1
  Production?/1 -> Product/2
  Product/1 -> Product2/2
  Sell Price to Utility (EUR)/1 -> Product2/1
  Product1/1 -> Product3/1
  Cost per kWh from Utility (EUR)/1 -> Product3/2
  Product3/1 -> Add/2
  Product2/1 -> Add/1
  Add/1 -> Result EUR/1

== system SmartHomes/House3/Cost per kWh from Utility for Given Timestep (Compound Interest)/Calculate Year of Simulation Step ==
  Digital Clock : DigitalClock
  Fcn : Fcn  Expr=floor(u/8760)
  Out1 : Outport
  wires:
  Fcn/1 -> Out1/1
  Digital Clock/1 -> Fcn/1

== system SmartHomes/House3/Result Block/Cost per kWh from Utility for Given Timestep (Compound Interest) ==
  Calculate Year of Simulation Step : Subsystem
  Compound Interest for Cost per kWh from Utility (EUR) : Fcn  Expr=u(2) * (1 + u(3) / 100) ^ u(1)
  Mux1 : Mux  Inputs=3
  annualChangeOfCostPerKwhFromUtility : Constant  Value=annualChangeOfCostPerKwhFromUtility
  costPerKwhFromUtility : Constant  Value=costPerKwhFromUtility
  Cost per kWh from Utility at Timestep : Outport
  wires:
  Mux1/1 -> Compound Interest for Cost per kWh from Utility (EUR)/1
  annualChangeOfCostPerKwhFromUtility/1 -> Mux1/3
  Calculate Year of Simulation Step/1(Out1) -> Mux1/1
  Compound Interest for Cost per kWh from Utility (EUR)/1 -> Cost per kWh from Utility at Timestep/1
  costPerKwhFromUtility/1 -> Mux1/2

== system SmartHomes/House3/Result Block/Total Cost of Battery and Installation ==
  Add : Sum
  Constant : Constant  Value=-1
  Divide : Product  Inputs=*/
  Number of Houses : Constant  Value=numberOfHouses
  Product : Product
  Product1 : Product
  batteryCostPerKwh : Constant  Value=batteryCostPerKwh
  "batterySize " : Constant  Value=batterySize
  oneTimeCost : Constant  Value=oneTimeCost
  Total Cost of Battery and Installation : Outport
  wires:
  Constant/1 -> Product/1
  oneTimeCost/1 -> Add/1
  Number of Houses/1 -> Divide/2
  Add/1 -> Divide/1
  Divide/1 -> Product/2
  "batterySize "/1 -> Product1/2
  Product/1 -> Total Cost of Battery and Installation/1
  batteryCostPerKwh/1 -> Product1/1
  Product1/1 -> Add/2

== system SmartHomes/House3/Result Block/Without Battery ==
  Effective Consumption / Production (kWh) : Inport
  Cost per kWh from Utility (EUR) : Inport  Port=2
  Sell Price to Utility (EUR) : Inport  Port=3
  Add : Sum
  Consumption? : simulink/Logic and Bit Operations/Compare To Zero  relop=<  OutDataTypeStr=boolean
  Product{,1..3} (4 alike) : Product
  Production? : simulink/Logic and Bit Operations/Compare To Zero  relop=>=  OutDataTypeStr=boolean
  Result EUR : Outport
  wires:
  Effective Consumption / Production (kWh)/1 -> Product/1, Product1/2, Consumption?/1, Production?/1
  Consumption?/1 -> Product1/1
  Production?/1 -> Product/2
  Product/1 -> Product2/2
  Sell Price to Utility (EUR)/1 -> Product2/1
  Product1/1 -> Product3/1
  Cost per kWh from Utility (EUR)/1 -> Product3/2
  Product3/1 -> Add/2
  Product2/1 -> Add/1
  Add/1 -> Result EUR/1

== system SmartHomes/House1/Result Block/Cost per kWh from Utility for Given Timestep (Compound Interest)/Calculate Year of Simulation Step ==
  Digital Clock : DigitalClock
  Fcn : Fcn  Expr=floor(u/8760)
  Out1 : Outport
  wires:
  Fcn/1 -> Out1/1
  Digital Clock/1 -> Fcn/1

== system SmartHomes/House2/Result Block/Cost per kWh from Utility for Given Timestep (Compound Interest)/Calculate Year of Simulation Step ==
  Digital Clock : DigitalClock
  Fcn : Fcn  Expr=floor(u/8760)
  Out1 : Outport
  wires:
  Fcn/1 -> Out1/1
  Digital Clock/1 -> Fcn/1

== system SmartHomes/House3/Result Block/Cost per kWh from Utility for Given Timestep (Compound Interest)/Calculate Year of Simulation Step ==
  Digital Clock : DigitalClock
  Fcn : Fcn  Expr=floor(u/8760)
  Out1 : Outport
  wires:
  Fcn/1 -> Out1/1
  Digital Clock/1 -> Fcn/1

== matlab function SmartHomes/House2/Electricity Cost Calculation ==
function [gridsaleAmount, cost]  = costCalculation(kWh, batteryStatus, buyPrice, sellPrice, internalSellPrice, internalBuyPrice)


cost = zeros(numel(batteryStatus)/3 , 1);
gridsaleAmount = zeros(numel(batteryStatus)/3 , 1);


for i = 1:numel(cost)
    
    %Production?
    
    if (kWh >= 0)
        
        cost(i) = kWh * sellPrice * batteryStatus((i-1)*3+1) + kWh * internalSellPrice * (batteryStatus((i-1)*3+2)+batteryStatus((i-1)*3+3));
        gridsaleAmount(i) = batteryStatus((i-1)*3+1);
        
    %Consumption?
    
    else
        
        cost(i) = kWh * buyPrice * batteryStatus((i-1)*3+3) + kWh * internalBuyPrice * (batteryStatus((i-1)*3+1)+batteryStatus((i-1)*3+2));
        gridsaleAmount(i) = 0;
        
    end
    
end

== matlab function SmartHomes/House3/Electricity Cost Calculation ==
function [gridsaleAmount, cost]  = costCalculation(kWh, batteryStatus, buyPrice, sellPrice, internalSellPrice, internalBuyPrice)


cost = zeros(numel(batteryStatus)/3 , 1);
gridsaleAmount = zeros(numel(batteryStatus)/3 , 1);


for i = 1:numel(cost)
    
    %Production?
    
    if (kWh >= 0)
        
        cost(i) = kWh * sellPrice * batteryStatus((i-1)*3+1) + kWh * internalSellPrice * (batteryStatus((i-1)*3+2)+batteryStatus((i-1)*3+3));
        gridsaleAmount(i) = batteryStatus((i-1)*3+1);
        
    %Consumption?
    
    else
        
        cost(i) = kWh * buyPrice * batteryStatus((i-1)*3+3) + kWh * internalBuyPrice * (batteryStatus((i-1)*3+1)+batteryStatus((i-1)*3+2));
        gridsaleAmount(i) = 0;
        
    end
    
end

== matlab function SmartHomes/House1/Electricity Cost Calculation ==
function [gridsaleAmount, cost]  = costCalculation(kWh, batteryStatus, buyPrice, sellPrice, internalSellPrice, internalBuyPrice)


cost = zeros(numel(batteryStatus)/3 , 1);
gridsaleAmount = zeros(numel(batteryStatus)/3 , 1);


for i = 1:numel(cost)
    
    %Production?
    
    if (kWh >= 0)
        
        cost(i) = kWh * sellPrice * batteryStatus((i-1)*3+1) + kWh * internalSellPrice * (batteryStatus((i-1)*3+2)+batteryStatus((i-1)*3+3));
        gridsaleAmount(i) = batteryStatus((i-1)*3+1);
        
    %Consumption?
    
    else
        
        cost(i) = kWh * buyPrice * batteryStatus((i-1)*3+3) + kWh * internalBuyPrice * (batteryStatus((i-1)*3+1)+batteryStatus((i-1)*3+2));
        gridsaleAmount(i) = 0;
        
    end
    
end

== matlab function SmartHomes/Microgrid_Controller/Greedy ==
function [p1,p2,p3]  = fcn(Consumption, Production, currentBatteryCharge, batterySize)
%fcn computes ???
%   Detailed desciription

p1 = 0;
p2 = 1;
p3 = 0;

Consumption = -Consumption;

% "Status" = aktueller Füllstand
% "Size" = Größe der Batterie in kWh

%Energie verkaufen
% Heißt "Strom muss an das externe Netz verkauft werden, falls die Batterie
% voll ist"?
if (currentBatteryCharge >= batterySize && Production ~= 0 && Consumption < Production)
    
    p2 = Consumption / Production;
    p1 = 1 - p2;
    
end

%Energie einkaufen
if (currentBatteryCharge <= 0 && Consumption ~= 0 && Consumption > Production)
    
    p2 = Production / Consumption;
    p3 = 1 - p2;
    
end

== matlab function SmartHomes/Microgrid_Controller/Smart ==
function [p1,p2,p3]  = fcn(Consumption, Production, currentBatteryCharge, batterySize)
%fcn computes ???
%   Detailed desciription

p1 = 0;
p2 = 1;
p3 = 0;

smart = 0.3;

Consumption = -Consumption;

% "Status" = aktueller Füllstand
% "Size" = Größe der Batterie in kWh

%Energie verkaufen
% Heißt "Strom muss an das externe Netz verkauft werden, falls die Batterie
% voll ist"?
if (currentBatteryCharge >= batterySize && Production ~= 0 && Consumption < Production)
    
    p2 = Consumption / Production;
    p1 = 1 - p2;
    
end

%Energie einkaufen
if (currentBatteryCharge <= batterySize * 0.3 && Consumption ~= 0 && Consumption > Production)
    
    p2 = Production / Consumption;
    p3 = 1 - p2;
    
end
